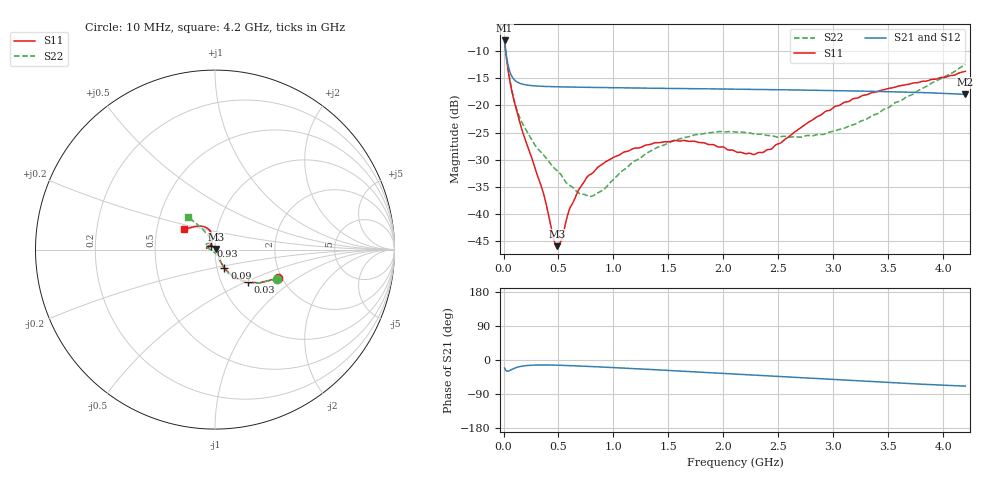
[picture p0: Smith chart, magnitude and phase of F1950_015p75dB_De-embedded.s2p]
! Integrated Device Technology
! Corporate Headquarters
! 6024 Silver Creek Valley Road
! San Jose, CA 95138  USA
! Phone:  1-408-284-8200
! Toll Free:  1-800-223-1366
! Webpage:  http://www.idt.com/
! Timing and RF Division
! 515 Groton Road, Suite 102
! Westford, MA 01886-6024
! Device:  F1950
! Description: 7-bit 0.25 dB Digital Step Attenuator
! Frequency:  150.0 -  4000.00 MHz
! Package:  4x4 mm Thin QFN Plastic Package: 24 pin
! Ports:  2 RF, 12 DC
!  Pin  1  = D0
!  Pin  2  = VDD
!  Pin  3  = Vmode
!  Pin  4  = GND
!  Pin  5  = RF1  =  Port 1
!  Pin  6  = GND
!  Pin  7  = GND
!  Pin  8  = GND
!  Pin  9  = GND
!  Pin 10  = GND
!  Pin 11  = GND
!  Pin 12  = GND
!  Pin 13  = GND
!  Pin 14  = RF2  =  Port 2
!  Pin 15  = GND
!  Pin 16  = LE
!  Pin 17  = CLK
!  Pin 18  = DATE
!  Pin 19  = D6
!  Pin 20  = D5
!  Pin 21  = D4
!  Pin 22  = D3
!  Pin 23  = D2
!  Pin 24  = D1
! State:  63
! Atten State:  15.75 dB
! Voltage:  +5.00 Volts
! Current:  Not Measured mA
! Data:  The device was measured on a the F195X evaluation board which has
!  individual transmission lines to the RF pins.  Data was collected
!  using a calibrated network analyzer.  The evaluation board was
!  de-embedded using a TRL calibration technique.
!  The reference plane is the edge of the package pin.
! Misc:  Board 2019
!  Action Tracker AT0250
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# GHz S dB R 50
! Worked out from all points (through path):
!   420 points, 10 MHz to 4.2 GHz, reference 50 ohm
!   highest |S21| = -8.05 dB at 10 MHz (marker M1); lowest = -18.0 dB at 4.2 GHz (marker M2)
!   group delay of S21, straight-line fit = 39.7 ps
!   lowest |S11| = -45.9 dB at 490 MHz (marker M3), VSWR 1.01, Z = 50.4 + j0.34 ohm
!   |S11| at or under -10 dB: 18.9 MHz to end of sweep
!   |S22| runs from -36.8 to -8.3 dB; largest |S21 - S12| = 0.00021
!   S11 on the Smith chart (normalised r, x): 10 MHz: 1.90, -0.71; 30 MHz: 1.33, -0.51; 90 MHz: 1.09, -0.23; 930 MHz: 0.95, +0.04; 4.2 GHz: 0.69, +0.16
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0.01  -8.31 -24.5  -8.05 -21.3  -8.05 -21.3  -8.33 -24.9
0.03  -11.82 -44.7  -11.34 -29.3  -11.34 -29.3  -11.71 -45.3
0.09  -18.68 -63.0  -15.10 -22.8  -15.10 -22.8  -18.49 -62.2
0.15  -23.29 -64.2  -15.96 -17.2  -15.96 -17.2  -22.36 -65.9
0.26  -29.86 -56.4  -16.38 -13.7  -16.38 -13.7  -26.45 -67.6
0.36  -36.00 -42.0  -16.51 -13.1  -16.51 -13.1  -29.03 -70.4
0.46  -44.94 5.1  -16.57 -13.5  -16.57 -13.5  -31.54 -75.1
0.49  -45.92 41.9  -16.59 -13.7  -16.59 -13.7  -32.07 -77.9
0.53  -44.57 77.7  -16.61 -14.1  -16.60 -14.1  -32.98 -79.3
0.6  -39.10 108.0  -16.63 -14.8  -16.63 -14.8  -34.73 -90.1
0.71  -34.79 122.8  -16.67 -16.1  -16.67 -16.1  -36.33 -109.5
0.8  -32.61 130.2  -16.70 -17.3  -16.69 -17.3  -36.74 -131.2
0.93  -30.37 139.2  -16.73 -19.1  -16.73 -19.1  -35.15 -159.0
1.17  -28.04 152.0  -16.80 -22.5  -16.80 -22.5  -30.54 176.1
1.41  -26.87 163.1  -16.86 -26.2  -16.86 -26.2  -27.64 165.9
1.73  -26.59 170.4  -16.93 -31.1  -16.93 -31.1  -25.47 156.7
2.11  -28.51 159.6  -17.03 -37.2  -17.02 -37.2  -24.92 147.0
2.43  -28.08 123.1  -17.11 -42.2  -17.11 -42.2  -25.57 136.5
2.81  -22.68 102.1  -17.22 -48.5  -17.21 -48.5  -25.60 120.6
3.1  -19.42 105.0  -17.32 -53.2  -17.31 -53.3  -24.20 115.5
3.51  -16.85 116.6  -17.49 -59.6  -17.48 -59.7  -20.31 117.1
4.2  -13.72 146.9  -17.99 -68.9  -17.98 -69.0  -12.50 129.4
